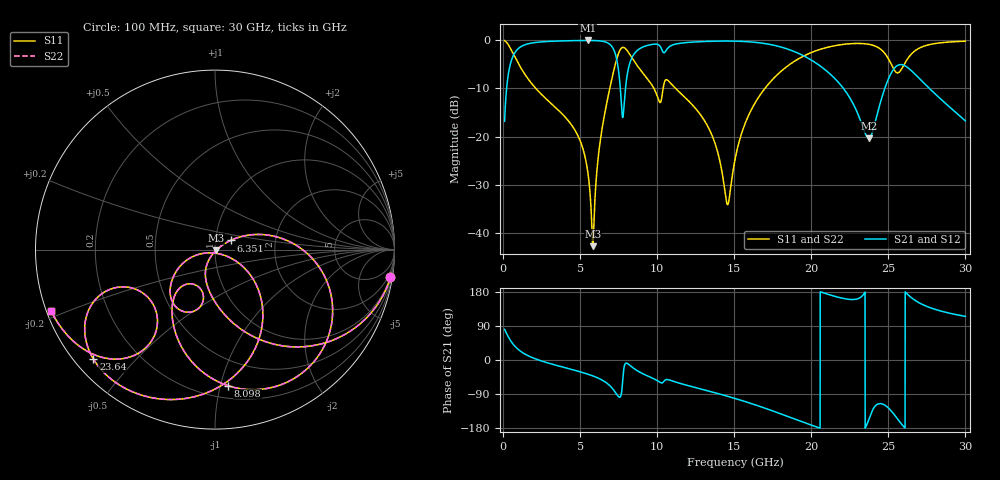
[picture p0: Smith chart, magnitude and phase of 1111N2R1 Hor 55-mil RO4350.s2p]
# GHz S MA R 50
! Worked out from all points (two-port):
!   3201 points, 100 MHz to 30 GHz, reference 50 ohm
!   highest |S21| = -0.06 dB at 5.501 GHz (marker M1); lowest = -20.4 dB at 23.73 GHz (marker M2)
!   |S21| within 3 dB of the highest: 683.8 MHz to 7.303 GHz (6.619 GHz wide, 166 % of centre); 8.461 GHz to 19.38 GHz (10.92 GHz wide, 78.5 % of centre)
!   lowest |S11| = -42.8 dB at 5.828 GHz (marker M3), VSWR 1.01, Z = 50.5 - j0.505 ohm
!   |S11| at or under -10 dB: 2.121 GHz to 6.926 GHz (4.805 GHz wide, 106 % of centre); 9.785 GHz to 10.39 GHz (602.6 MHz wide, 5.97 % of centre); 11.19 GHz to 16.99 GHz (5.802 GHz wide, 41.2 % of centre)
!   |S22| runs from -42.8 to -0.1 dB; largest |S21 - S12| = 0
!   S11 on the Smith chart (normalised r, x): 100 MHz: 1, -13; 6.351 GHz: 1.18, +0.12; 8.098 GHz: 0.29, -1.05; 23.64 GHz: 0.05, -0.38; 30 GHz: 0.01, -0.18
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0.1  0.9895 -9.0  0.1439 81.0  0.1439 81.0  0.9895 -9.0
0.5765313  0.7669 -44.2  0.641 45.8  0.641 45.8  0.7669 -44.2
1.585656  0.4041 -77.8  0.9134 12.1  0.9134 12.1  0.4041 -77.8
5.089563  0.08283 -119.6  0.9922 -32.2  0.9922 -32.2  0.08283 -119.6
5.500687  0.04245 -120.3  0.9932 -37.4  0.9932 -37.4  0.04245 -120.3
5.827719  0.007271 -43.5  0.9921 -42.1  0.9921 -42.1  0.007271 -43.5
6.350969  0.1009 30.5  0.9799 -51.4  0.9799 -51.4  0.1009 30.5
7.070437  0.4034 7.3  0.855 -74.0  0.855 -74.0  0.4034 7.3
7.50025  0.7344 -26.8  0.4733 -97.0  0.4733 -97.0  0.7344 -26.8
7.771219  0.8421 -56.0  0.1578 -49.9  0.1578 -49.9  0.8421 -56.0
8.09825  0.7611 -84.6  0.4773 -9.9  0.4773 -9.9  0.7611 -84.6
10.06978  0.2453 -128.6  0.8977 -56.1  0.8977 -56.1  0.2453 -128.6
12.92897  0.1582 -160.4  0.9667 -77.5  0.9667 -77.5  0.1582 -160.4
14.55478  0.0197 -100.8  0.9789 -95.6  0.9789 -95.6  0.0197 -100.8
15.05  0.0575 -32.2  0.9767 -101.5  0.9767 -101.5  0.0575 -32.2
16.77859  0.2846 -39.0  0.9327 -124.1  0.9327 -124.1  0.2846 -39.0
20.03956  0.748 -86.0  0.6161 -172.4  0.6161 -172.4  0.748 -86.0
23.63691  0.9114 -138.0  0.0978 -167.5  0.0978 -167.5  0.9114 -138.0
23.73034  0.9063 -139.5  0.0956 -157.5  0.0956 -157.5  0.9063 -139.5
25.01978  0.635 -159.2  0.4009 -127.2  0.4009 -127.2  0.635 -159.2
25.98219  0.5432 -126.6  0.5512 -175.2  0.5512 -175.2  0.5432 -126.6
30  0.9752 -159.4  0.1453 115.1  0.1453 115.1  0.9752 -159.4
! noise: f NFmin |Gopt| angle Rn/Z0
0.1  0.001761  0.9048  3.031  0.004055
3.417  0.01124  0.5343  27.52  0.004045
6.743  0.05907  0.8014  47.92  0.05162
10.06  0.1137  0.8484  69.76  0.1078
13.39  0.0651  0.6894  89.66  0.02119
16.7  0.08229  0.7006  106.1  0.0205
20.03  0.1512  0.8006  122.2  0.03821
23.35  1.195  0.968  139.3  1.04
26.67  0.4425  0.9054  153.6  0.05606
30  0.5018  0.9152  166.1  0.02177
